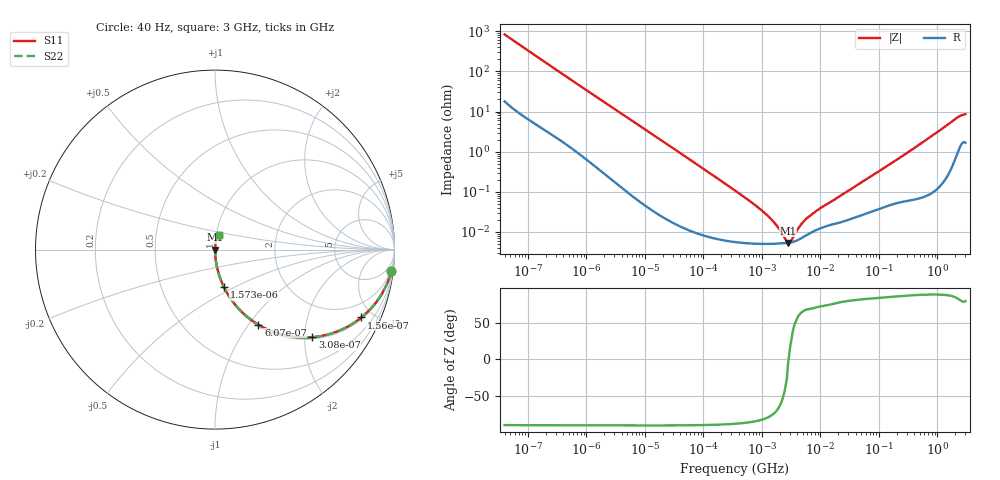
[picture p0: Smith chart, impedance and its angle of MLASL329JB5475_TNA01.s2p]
! MLASL329JB5475_TNA01  S-PARAMETER MODEL  ( General Type )
! Model Generated by TAIYO YUDEN Corporation (http://www.ty-top.com)
! Version 2.0
! TAIYO YUDEN Control No. 100817
! Copyright(c) 2009 TAIYO YUDEN CO.,LTD. All Rights Reserved.
! Product Description (link to TY-COMPAS)
! https://ds.yuden.co.jp/TYCOMPAS/or/detail?pn=MLASL329JB5475KTNA01&u=M
! Products Name : Multilayer Ceramic Capacitors
! Characteristics :
!  Capacitance : 4.7 uF , Rated Voltage : 10V , TCC : B / X5R
!  Case Size : 3.2 x 2.5 / 0.126 x 0.098 [mm/inch] , Thickness : 0.85 / 0.033 [mm/inch]
!  (Conditions: Temperature = 25 degC , DC Bias Current/Voltage = 0A / 0V)
! External Node Assignments :
!  1  o---| |---o  2
! GND o---------o GND
! Frequency Range : 40Hz  -  3GHz  [ 401 STEP ]
# MHz S RI R 50
! Freq[MHz].  S11 Real  S11 Imag  S21 Real  S21 Imag  S12 Real  S12 Imag  S22 Real  S22 Imag
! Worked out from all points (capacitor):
!   401 points, 40 Hz to 3 GHz, reference 50 ohm
!   read as one part in series: C = 4.79 uF near 44 Hz
!   lowest |Z| = 5.35 mohm at 2.788 MHz (marker M1)
!   series resonance near 2.854 MHz, so ESL is about 650 pH
!   S11 on the Smith chart (normalised r, x): 40 Hz: 1, -17; 156 Hz: 1.08, -4.27; 308 Hz: 1.04, -2.18; 607 Hz: 1.02, -1.11; 1.573 kHz: 1.01, -0.44; 3 GHz: 1.03, +0.17
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4e-05  0.9833 -0.1178  0.0167 0.1178  0.0167 0.1178  0.9833 -0.1178
8.3e-05  0.9374 -0.2328  0.0626 0.2328  0.0626 0.2328  0.9374 -0.2328
0.000156  0.8156 -0.378  0.1844 0.378  0.1844 0.378  0.8156 -0.378
0.000308  0.5418 -0.4881  0.4582 0.4881  0.4582 0.4881  0.5418 -0.4881
0.000422  0.3911 -0.4779  0.6089 0.4779  0.6089 0.4779  0.3911 -0.4779
0.000607  0.2414 -0.4181  0.7586 0.4181  0.7586 0.4181  0.2414 -0.4181
0.000834  0.1471 -0.3447  0.8529 0.3447  0.8529 0.3447  0.1471 -0.3447
0.001573  0.0492 -0.2079  0.9508 0.2079  0.9508 0.2079  0.0492 -0.2079
0.004462  0.00744 -0.0793  0.9926 0.0793  0.9926 0.0793  0.00744 -0.0793
0.017386  0.000715 -0.0211  0.9993 0.0211  0.9993 0.0211  0.000715 -0.0211
0.362475  5.68e-05 -0.00103  0.9999 0.00103  0.9999 0.00103  5.68e-05 -0.00103
1.075925  5.06e-05 -0.000308  0.9999 0.000308  0.9999 0.000308  5.06e-05 -0.000308
1.477731  5.08e-05 -0.000193  0.9999 0.000193  0.9999 0.000193  5.08e-05 -0.000193
2.123718  5.23e-05 -8.61e-05  0.9999 8.61e-05  0.9999 8.61e-05  5.23e-05 -8.61e-05
2.78755  5.32e-05 -5.74e-06  0.9999 5.74e-06  0.9999 5.74e-06  5.32e-05 -5.74e-06
3.496721  5.74e-05 5.47e-05  0.9999 -5.47e-05  0.9999 -5.47e-05  5.74e-05 5.47e-05
3.828567  6.04e-05 7.74e-05  0.9999 -7.74e-05  0.9999 -7.74e-05  6.04e-05 7.74e-05
5.258354  7.68e-05 0.000171  0.9999 -0.000171  0.9999 -0.000171  7.68e-05 0.000171
7.222098  9.97e-05 0.000259  0.9999 -0.000259  0.9999 -0.000259  9.97e-05 0.000259
150.5692  0.000485 0.00477  0.9995 -0.00477  0.9995 -0.00477  0.000485 0.00477
2087.469  0.0119 0.0661  0.9881 -0.0661  0.9881 -0.0661  0.0119 0.0661
3000  0.0232 0.0816  0.9768 -0.0816  0.9768 -0.0816  0.0232 0.0816
